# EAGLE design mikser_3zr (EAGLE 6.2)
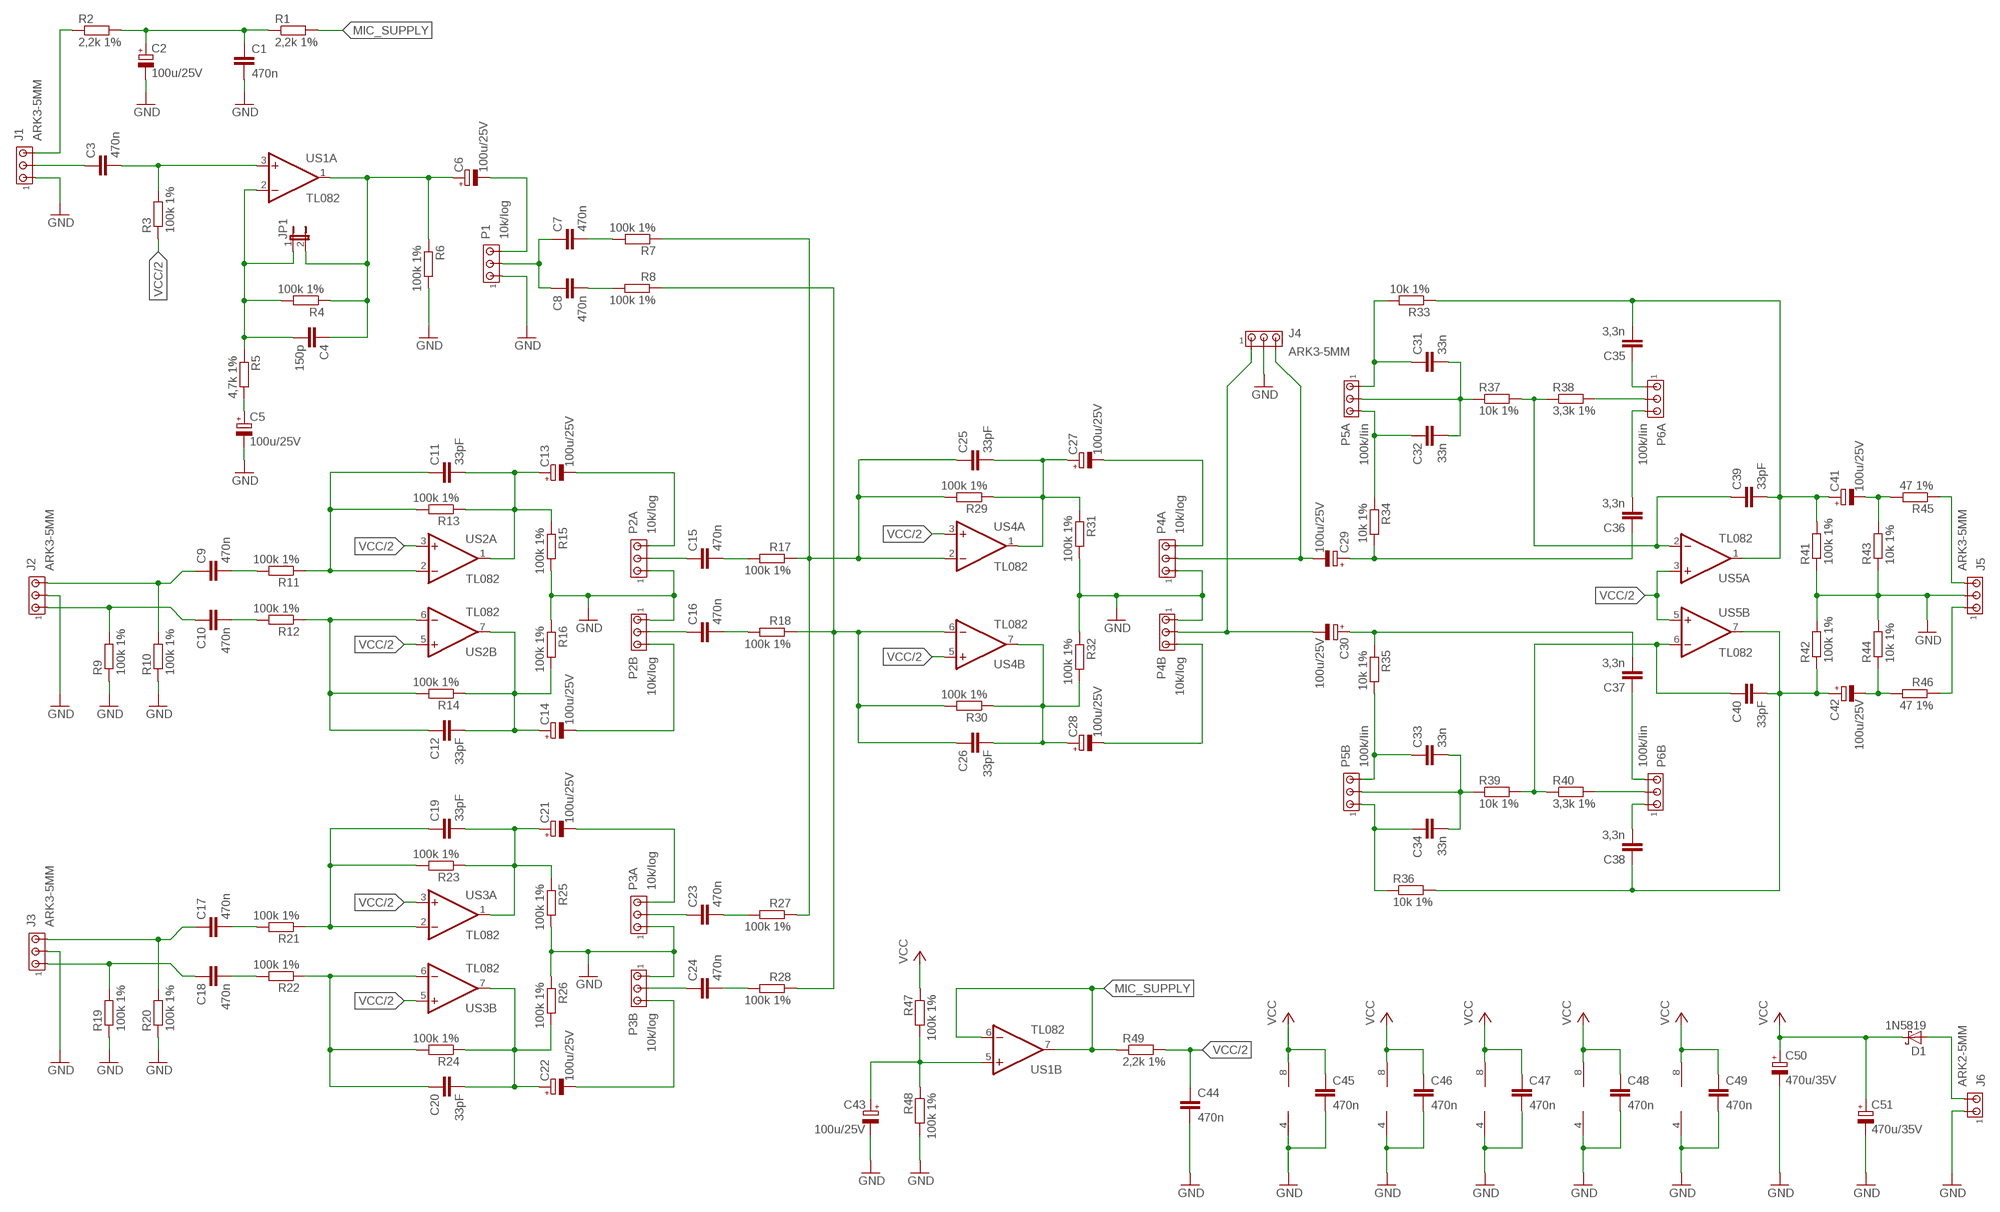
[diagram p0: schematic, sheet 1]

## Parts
C1  470n  C-EU050-055X075  [C050-055X075]
C2  100u/25V  CPOL-EUE2.5-6  [E2,5-6]
C3  470n  C-EU050-055X075  [C050-055X075]
C4  150p  C-EU050-025X075  [C050-025X075]
C5  100u/25V  CPOL-EUE2.5-6  [E2,5-6]
C6  100u/25V  CPOL-EUE2.5-6  [E2,5-6]
C7  470n  C-EU050-055X075  [C050-055X075]
C8  470n  C-EU050-055X075  [C050-055X075]
C9  470n  C-EU050-055X075  [C050-055X075]
C10  470n  C-EU050-055X075  [C050-055X075]
C11  33pF  C-EU050-025X075  [C050-025X075]
C12  33pF  C-EU050-025X075  [C050-025X075]
C13  100u/25V  CPOL-EUE2.5-6  [E2,5-6]
C14  100u/25V  CPOL-EUE2.5-6  [E2,5-6]
C15  470n  C-EU050-055X075  [C050-055X075]
C16  470n  C-EU050-055X075  [C050-055X075]
C17  470n  C-EU050-055X075  [C050-055X075]
C18  470n  C-EU050-055X075  [C050-055X075]
C19  33pF  C-EU050-025X075  [C050-025X075]
C20  33pF  C-EU050-025X075  [C050-025X075]
C21  100u/25V  CPOL-EUE2.5-6  [E2,5-6]
C22  100u/25V  CPOL-EUE2.5-6  [E2,5-6]
C23  470n  C-EU050-055X075  [C050-055X075]
C24  470n  C-EU050-055X075  [C050-055X075]
C25  33pF  C-EU050-025X075  [C050-025X075]
C26  33pF  C-EU050-025X075  [C050-025X075]
C27  100u/25V  CPOL-EUE2.5-6  [E2,5-6]
C28  100u/25V  CPOL-EUE2.5-6  [E2,5-6]
C29  100u/25V  CPOL-EUE2.5-6  [E2,5-6]
C30  100u/25V  CPOL-EUE2.5-6  [E2,5-6]
C31  33n  C-EU050-025X075  [C050-025X075]
C32  33n  C-EU050-025X075  [C050-025X075]
C33  33n  C-EU050-025X075  [C050-025X075]
C34  33n  C-EU050-025X075  [C050-025X075]
C35  3,3n  C-EU050-025X075  [C050-025X075]
C36  3,3n  C-EU050-025X075  [C050-025X075]
C37  3,3n  C-EU050-025X075  [C050-025X075]
C38  3,3n  C-EU050-025X075  [C050-025X075]
C39  33pF  C-EU050-025X075  [C050-025X075]
C40  33pF  C-EU050-025X075  [C050-025X075]
C41  100u/25V  CPOL-EUE2.5-6  [E2,5-6]
C42  100u/25V  CPOL-EUE2.5-6  [E2,5-6]
C43  100u/25V  CPOL-EUE2.5-6  [E2,5-6]
C44  470n  C-EU050-055X075  [C050-055X075]
C45  470n  C-EU050-055X075  [C050-055X075]
C46  470n  C-EU050-055X075  [C050-055X075]
C47  470n  C-EU050-055X075  [C050-055X075]
C48  470n  C-EU050-055X075  [C050-055X075]
C49  470n  C-EU050-055X075  [C050-055X075]
C50  470u/35V  CPOL-EUE5-10.5  [E5-10,5]
C51  470u/35V  CPOL-EUE5-10.5  [E5-10,5]
D1  1N5819  1N5817-B  [DO41-7.6]
J1  ARK3-5MM  [3PIN-5MM]
J2  ARK3-5MM  [3PIN-5MM]
J3  ARK3-5MM  [3PIN-5MM]
J4  ARK3-5MM  [3PIN-5MM]
J5  ARK3-5MM  [3PIN-5MM]
J6  ARK2-5MM  [2PIN-5MM]
JP1  JP1E  [JP1]
P1  10k/log  ARK3-5MM-WASKI  [3PIN-5M-WASKI]
P2A  10k/log  ARK3-5MM-WASKI  [3PIN-5M-WASKI]
P2B  10k/log  ARK3-5MM-WASKI  [3PIN-5M-WASKI]
P3A  10k/log  ARK3-5MM-WASKI  [3PIN-5M-WASKI]
P3B  10k/log  ARK3-5MM-WASKI  [3PIN-5M-WASKI]
P4A  10k/log  ARK3-5MM-WASKI  [3PIN-5M-WASKI]
P4B  10k/log  ARK3-5MM-WASKI  [3PIN-5M-WASKI]
P5A  100k/lin  ARK3-5MM-WASKI  [3PIN-5M-WASKI]
P5B  100k/lin  ARK3-5MM-WASKI  [3PIN-5M-WASKI]
P6A  100k/lin  ARK3-5MM-WASKI  [3PIN-5M-WASKI]
P6B  100k/lin  ARK3-5MM-WASKI  [3PIN-5M-WASKI]
R1  2,2k 1%  R-EU_0207/7  [0207/7]
R2  2,2k 1%  R-EU_0207/7  [0207/7]
R3  100k 1%  R-EU_0207/7  [0207/7]
R4  100k 1%  R-EU_0207/7  [0207/7]
R5  4,7k 1%  R-EU_0207/7  [0207/7]
R6  100k 1%  R-EU_0207/7  [0207/7]
R7  100k 1%  R-EU_0207/7  [0207/7]
R8  100k 1%  R-EU_0207/7  [0207/7]
R9  100k 1%  R-EU_0207/7  [0207/7]
R10  100k 1%  R-EU_0207/7  [0207/7]
R11  100k 1%  R-EU_0207/7  [0207/7]
R12  100k 1%  R-EU_0207/7  [0207/7]
R13  100k 1%  R-EU_0207/7  [0207/7]
R14  100k 1%  R-EU_0207/7  [0207/7]
R15  100k 1%  R-EU_0207/7  [0207/7]
R16  100k 1%  R-EU_0207/7  [0207/7]
R17  100k 1%  R-EU_0207/7  [0207/7]
R18  100k 1%  R-EU_0207/7  [0207/7]
R19  100k 1%  R-EU_0207/7  [0207/7]
R20  100k 1%  R-EU_0207/7  [0207/7]
R21  100k 1%  R-EU_0207/7  [0207/7]
R22  100k 1%  R-EU_0207/7  [0207/7]
R23  100k 1%  R-EU_0207/7  [0207/7]
R24  100k 1%  R-EU_0207/7  [0207/7]
R25  100k 1%  R-EU_0207/7  [0207/7]
R26  100k 1%  R-EU_0207/7  [0207/7]
R27  100k 1%  R-EU_0207/7  [0207/7]
R28  100k 1%  R-EU_0207/7  [0207/7]
R29  100k 1%  R-EU_0207/7  [0207/7]
R30  100k 1%  R-EU_0207/7  [0207/7]
R31  100k 1%  R-EU_0207/7  [0207/7]
R32  100k 1%  R-EU_0207/7  [0207/7]
R33  10k 1%  R-EU_0207/7  [0207/7]
R34  10k 1%  R-EU_0207/7  [0207/7]
R35  10k 1%  R-EU_0207/7  [0207/7]
R36  10k 1%  R-EU_0207/7  [0207/7]
R37  10k 1%  R-EU_0207/7  [0207/7]
R38  3,3k 1%  R-EU_0207/7  [0207/7]
R39  10k 1%  R-EU_0207/7  [0207/7]
R40  3,3k 1%  R-EU_0207/7  [0207/7]
R41  100k 1%  R-EU_0207/7  [0207/7]
R42  100k 1%  R-EU_0207/7  [0207/7]
R43  10k 1%  R-EU_0207/7  [0207/7]
R44  10k 1%  R-EU_0207/7  [0207/7]
R45  47 1%  R-EU_0207/7  [0207/7]
R46  47 1%  R-EU_0207/7  [0207/7]
R47  100k 1%  R-EU_0207/7  [0207/7]
R48  100k 1%  R-EU_0207/7  [0207/7]
R49  2,2k 1%  R-EU_0207/7  [0207/7]
US1  TL082  TL082P  [DIL08]
US2  TL082  TL082P  [DIL08]
US3  TL082  TL082P  [DIL08]
US4  TL082  TL082P  [DIL08]
US5  TL082  TL082P  [DIL08]

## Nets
GND: C1.2 C2.- C5.- C43.- C44.2 C45.2 C46.2 C47.2 C48.2 C49.2 C50.- C51.- J1.P$1 J2.P$2 J3.P$2 J4.P$2 J5.P$2 J6.P$1 P1.P$1 P2A.P$1 P2B.P$1 P3A.P$1 P3B.P$1 P4A.P$1 P4B.P$1 R6.2 R9.1 R10.1 R15.2 R16.1 R19.1 R20.1 R25.2 R26.1 R31.2 R32.1 R41.1 R42.2 R43.1 R44.2 R48.2 US1.4(P:V-) US2.4(P:V-) US3.4(P:V-) US4.4(P:V-) US5.4(P:V-)
MIC_SUPPLY: R1.2 R49.1 US1.6(B:-IN) US1.7(B:OUT)
N$1: J1.P$3 R2.1
N$2: C1.1 C2.+ R1.1 R2.2
N$3: C3.1 J1.P$2
N$4: C3.2 R3.2 US1.3(A:+IN)
N$5: C5.+ R5.2
N$6: C4.2 JP1.1 R4.2 R5.1 US1.2(A:-IN)
N$7: C6.- P1.P$3
N$8: C4.1 C6.+ JP1.2 R4.1 R6.1 US1.1(A:OUT)
N$9: C7.1 C8.1 P1.P$2
N$10: C7.2 R7.2
N$11: C8.2 R8.2
N$12: C10.1 J2.P$1 R9.2
N$13: C9.1 J2.P$3 R10.2
N$14: C9.2 R11.2
N$15: C10.2 R12.2
N$16: C11.2 C13.+ R13.1 R15.1 US2.1(A:OUT)
N$17: C12.2 C14.+ R14.1 R16.2 US2.7(B:OUT)
N$18: C12.1 R12.1 R14.2 US2.6(B:-IN)
N$19: C11.1 R11.1 R13.2 US2.2(A:-IN)
N$20: C13.- P2A.P$3
N$21: C14.- P2B.P$3
N$22: C16.2 R18.2
N$23: C16.1 P2B.P$2
N$24: C15.1 P2A.P$2
N$25: C15.2 R17.2
N$26: C18.1 J3.P$1 R19.2
N$27: C17.1 J3.P$3 R20.2
N$28: C17.2 R21.2
N$29: C18.2 R22.2
N$30: C20.1 R22.1 R24.2 US3.6(B:-IN)
N$31: C19.1 R21.1 R23.2 US3.2(A:-IN)
N$32: C19.2 C21.+ R23.1 R25.1 US3.1(A:OUT)
N$33: C20.2 C22.+ R24.1 R26.2 US3.7(B:OUT)
N$34: C21.- P3A.P$3
N$35: C22.- P3B.P$3
N$36: C24.2 R28.2
N$37: C24.1 P3B.P$2
N$38: C23.1 P3A.P$2
N$39: C23.2 R27.2
N$40: C26.1 R8.1 R18.1 R28.1 R30.2 US4.6(B:-IN)
N$41: C25.1 R7.1 R17.1 R27.1 R29.2 US4.2(A:-IN)
N$42: C25.2 C27.+ R29.1 R31.1 US4.1(A:OUT)
N$43: C26.2 C28.+ R30.1 R32.2 US4.7(B:OUT)
N$44: C27.- P4A.P$3
N$45: C28.- P4B.P$3
N$46: C30.- J4.P$1 P4B.P$2
N$47: C29.- J4.P$3 P4A.P$2
N$48: C29.+ C36.1 R34.2
N$49: C30.+ C37.2 R35.1
N$50: C41.- R43.2 R45.2
N$51: C42.- R44.1 R46.2
N$52: C43.+ R47.2 R48.1 US1.5(B:+IN)
N$53: J5.P$1 R46.1
N$54: J5.P$3 R45.1
N$55: D1.A J6.P$2
N$58: C32.1 P5A.P$3 R34.1
N$59: C31.1 P5A.P$1 R33.2
N$60: C31.2 C32.2 P5A.P$2 R37.1
N$61: C39.1 R37.2 R38.1 US5.2(A:-IN)
N$62: P6A.P$2 R38.2
N$63: C35.2 C39.2 C41.+ R33.1 R41.2 US5.1(A:OUT)
N$65: C33.1 P5B.P$3 R35.2
N$66: C34.1 P5B.P$1 R36.1
N$67: C33.2 C34.2 P5B.P$2 R39.1
N$68: C38.1 C40.2 C42.+ R36.2 R42.1 US5.7(B:OUT)
N$69: C40.1 R39.2 R40.1 US5.6(B:-IN)
N$70: P6B.P$2 R40.2
N$76: C38.2 P6B.P$1
N$77: C37.1 P6B.P$3
N$78: C36.2 P6A.P$3
N$79: C35.1 P6A.P$1
VCC: C45.1 C46.1 C47.1 C48.1 C49.1 C50.+ C51.+ D1.C R47.1 US1.8(P:V+) US2.8(P:V+) US3.8(P:V+) US4.8(P:V+) US5.8(P:V+)
VCC/2: C44.1 R3.1 R49.2 US2.3(A:+IN) US2.5(B:+IN) US3.3(A:+IN) US3.5(B:+IN) US4.3(A:+IN) US4.5(B:+IN) US5.3(A:+IN) US5.5(B:+IN)

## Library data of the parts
C1 C3 C4 C7-C12 C15-C20 C23-C26 C31-C40 C44-C49 = rcl:C-EU: CAPACITOR, European symbol
C2 C5 C6 C13 C14 C21 C22 C27-C30 C41-C43 C50 C51 = rcl:CPOL-EU: POLARIZED CAPACITOR, European symbol
D1 = diode:1N581*: 1.0A SCHOTTKY BARRIER RECTIFIER
J1-J5 P1 P2A P2B P3A P3B P4A P4B P5A P5B P6A P6B = zlacza_futrzak:ARK3: ARK 3 Raster 5mm i 3,5mm
J6 = zlacza_futrzak:ARK2: ARK 2
JP1 = jumper:JP1E: JUMPER
R1-R49 = rcl:R-EU_: RESISTOR, European symbol
US1-US5 = linear:TL082: OP AMP

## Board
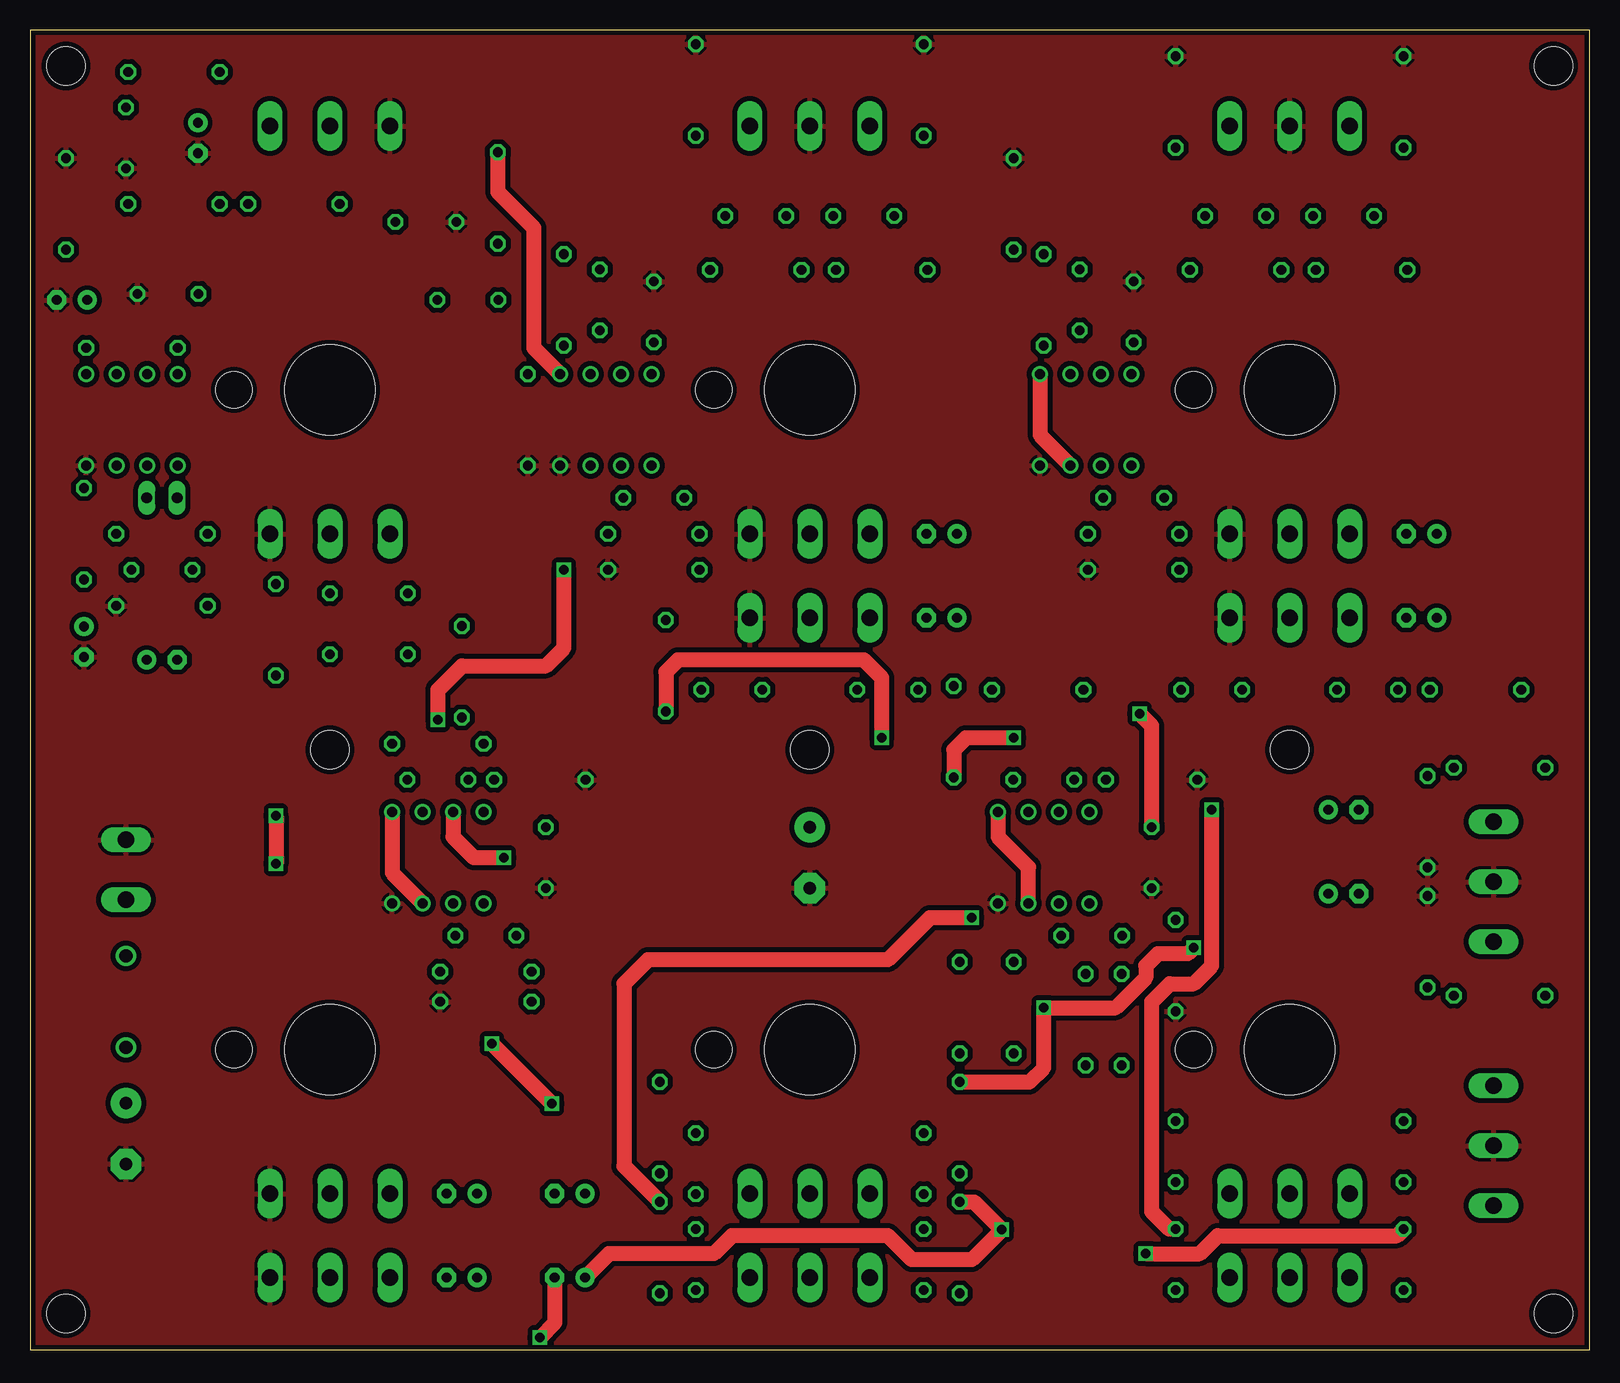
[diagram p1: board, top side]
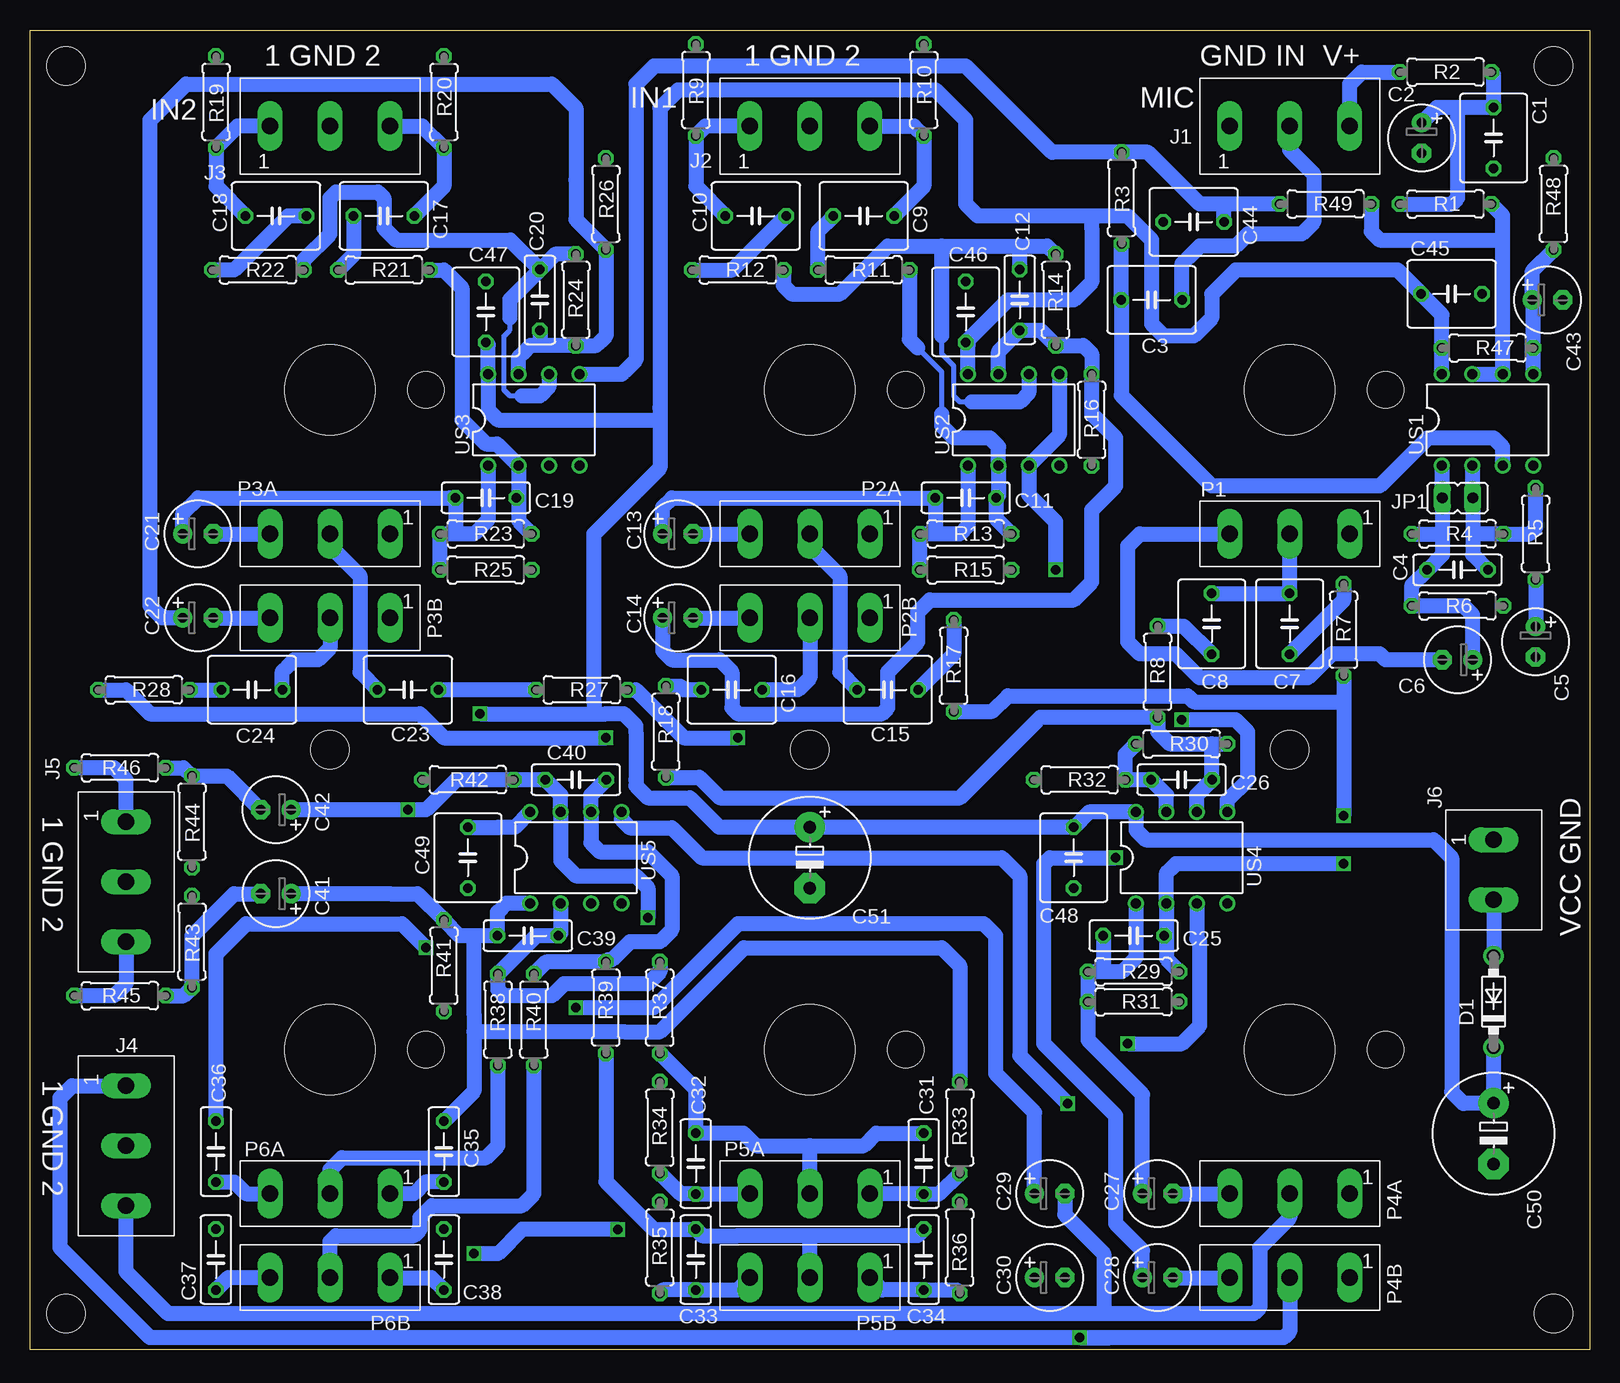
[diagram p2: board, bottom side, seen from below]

Size 130 x 110 mm. Coordinates in mm from the lower left corner, seen from the top.
Outline: 0,0 130,0 130,110 0,110 0,0
Copper layers (1*16): Top 0.035mm / dielectric 1.5mm / Bottom 0.035mm
Design rules: minimum track width 10mil, minimum drill 24mil, track to track 8mil, track to pad 8mil, pad to pad 8mil, via to via 8mil, smd to smd 8mil, copper to edge 10mil, drill to drill 8mil, minimum pad ring 10mil, minimum via ring 8mil, stop-mask expansion 4mil, vias tented up to drill 0mil, thermal gap 10mil
Holes 3.2 mm at 3,3 3,107 127,107 127,3 25,50 65,50 105,50
Holes 7.5 mm at 25,80 65,80 105,80 25,25 65,25 105,25
Holes 3 mm at 17,80 57,80 97,80 17,25 57,25 97,25

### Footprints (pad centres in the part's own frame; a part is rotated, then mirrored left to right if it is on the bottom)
C050-055X075 = drill 0.813 octagon: 1 -2.54,0; 2 2.54,0
E2,5-6 = drill 0.813 pad 1.6: + -1.27,0 | drill 0.813 pad 1.6 octagon: - 1.27,0
C050-025X075 = drill 0.813 octagon: 1 -2.54,0; 2 2.54,0
E5-10,5 = drill 1.016 pad 2.54: + -2.54,0 | drill 1.016 pad 2.54 octagon: - 2.54,0
DO41-7.6 = drill 1.1 pad 1.7: A 3.81,0; C -3.81,0
3PIN-5MM = drill 1.4 long: P$1 -5,0; P$2 0,0; P$3 5,0
2PIN-5MM = drill 1.4 long: P$1 -2.5,0; P$2 2.5,0
JP1 = drill 0.914 long: 1 0,-1.27; 2 0,1.27
3PIN-5M-WASKI = drill 1.4 long: P$1 -5,0; P$2 0,0; P$3 5,0
0207/7 = drill 0.813 octagon: 1 -3.81,0; 2 3.81,0
DIL08 = drill 0.813 pad 1.27: 1 -3.81,-3.81; 2 -1.27,-3.81; 3 1.27,-3.81; 4 3.81,-3.81; 5 3.81,3.81; 6 1.27,3.81; 7 -1.27,3.81; 8 -3.81,3.81

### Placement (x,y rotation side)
C1  8,101 270 bottom
C2  14,101 270 bottom
C3  36.5,87.5 180 bottom
C4  11,65 0 bottom
C5  4.5,59 270 bottom
C6  11,57.5 180 bottom
C7  25,60.5 270 bottom
C8  31.5,60.5 270 bottom
C9  60.5,94.5 180 bottom
C10  69.5,94.5 0 bottom
C11  52,71 180 bottom
C12  47.5,87.5 270 bottom
C13  76,68 0 bottom
C14  76,61 0 bottom
C15  58.5,55 0 bottom
C16  71.5,55 180 bottom
C17  100.5,94.5 180 bottom
C18  109.5,94.5 0 bottom
C19  92,71 180 bottom
C20  87.5,87.5 270 bottom
C21  116,68 0 bottom
C22  116,61 0 bottom
C23  98.5,55 0 bottom
C24  111.5,55 180 bottom
C25  38,34.5 180 bottom
C26  34,47.5 180 bottom
C27  36,13 0 bottom
C28  36,6 0 bottom
C29  45,13 0 bottom
C30  45,6 0 bottom
C31  55.5,15.5 90 bottom
C32  74.5,15.5 90 bottom
C33  74.5,7.5 90 bottom
C34  55.5,7.5 90 bottom
C35  95.5,16.5 90 bottom
C36  114.5,16.5 270 bottom
C37  114.5,7.5 90 bottom
C38  95.5,7.5 270 bottom
C39  88.5,34.5 180 bottom
C40  84.5,47.5 180 bottom
C41  109.5,38 180 bottom
C42  109.5,45 180 bottom
C43  3.5,87.5 0 bottom
C44  33,94 180 bottom
C45  11.5,88 0 bottom
C46  52,86.5 90 bottom
C47  92,86.5 90 bottom
C48  43,41 270 bottom
C49  93.5,41 270 bottom
C50  8,18 270 bottom
C51  65,41 270 bottom
D1  8,29 90 bottom
J1  25,102 0 bottom
J2  65,102 0 bottom
J3  105,102 0 bottom
J4  122,17 270 bottom
J5  122,39 270 bottom
J6  8,40 270 bottom
JP1  11,71 90 bottom
P1  25,68 180 bottom
P2A  65,68 180 bottom
P2B  65,61 180 bottom
P3A  105,68 180 bottom
P3B  105,61 180 bottom
P4A  25,13 180 bottom
P4B  25,6 180 bottom
P5A  65,13 180 bottom
P5B  65,6 180 bottom
P6A  105,13 180 bottom
P6B  105,6 180 bottom
R1  12,95.5 0 bottom
R2  12,106.5 0 bottom
R3  39,96 270 bottom
R4  11,68 0 bottom
R5  4.5,68 270 bottom
R6  11,62 0 bottom
R7  20.5,60 90 bottom
R8  36,56.5 90 bottom
R9  74.5,105 270 bottom
R10  55.5,105 270 bottom
R11  60.5,90 180 bottom
R12  71,90 180 bottom
R13  52,68 0 bottom
R14  44.5,87.5 90 bottom
R15  52,65 0 bottom
R16  41.5,77.5 90 bottom
R17  53,57 90 bottom
R18  77,51.5 90 bottom
R19  114.5,104 270 bottom
R20  95.5,104 270 bottom
R21  100.5,90 180 bottom
R22  111,90 180 bottom
R23  92,68 0 bottom
R24  84.5,87.5 90 bottom
R25  92,65 0 bottom
R26  82,95.5 270 bottom
R27  84,55 180 bottom
R28  120.5,55 0 bottom
R29  38,31.5 0 bottom
R30  34,50.5 0 bottom
R31  38,29 0 bottom
R32  42.5,47.5 0 bottom
R33  52.5,18.5 270 bottom
R34  77.5,18.5 90 bottom
R35  77.5,8.5 270 bottom
R36  52.5,8.5 90 bottom
R37  77.5,28.5 90 bottom
R38  91,27.5 270 bottom
R39  82,28.5 90 bottom
R40  88,27.5 270 bottom
R41  95.5,32 90 bottom
R42  93.5,47.5 180 bottom
R43  116.5,34 270 bottom
R44  116.5,44 270 bottom
R45  122.5,29.5 0 bottom
R46  122.5,48.5 0 bottom
R47  8.5,83.5 0 bottom
R48  3,95.5 90 bottom
R49  22,95.5 180 bottom
US1  8.5,77.5 0 bottom
US2  48,77.5 0 bottom
US3  88,77.5 0 bottom
US4  34,41 0 bottom
US5  84.5,41 0 bottom

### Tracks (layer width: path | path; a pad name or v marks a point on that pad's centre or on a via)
GND
  pour Top (isolate 0.406): 0,0 130,0 130,110 0,110
MIC_SUPPLY
  Bottom 1.27: US1.7 US1.6 7.23,92.5 | 7.23,92.5 7.23,94.54 R1.2 | R49.1 18.19,93.19 17.5,92.5 7.23,92.5
N$1
  Bottom 1.27: J1.P$3 20,105.5 19,106.5 R2.1
N$2
  Bottom 1.27: 11,103.54 C1.1 8,106.31 R2.2 | 11,103.54 12.73,103.54 C2.+ | R1.1 11.5,95.5 11,96 11,103.54
N$3
  Bottom 1.27: J1.P$2 25,100 23,98 23,94 24,93 28.5,93 29.5,92 32.5,92 33.5,91 33.96,90.54 C3.1
N$4
  Bottom 1.27: R3.2 39.04,92.15 C3.2 39.04,79.54 31.5,72 17.5,72 13.5,76 8,76 7.23,75.23 US1.3
N$5
  Bottom 1.27: R5.2 C5.+
N$6
  Bottom 1.27: US1.2 9.77,71.04 JP1.1 9.73,68 | 9.73,68 9.73,66.27 C4.2 | 9.73,68 R4.2 5,68 4.5,68.5 R5.1
N$7
  Bottom 1.27: C6.- 17,57.5 17.5,58 21.5,58 23,56.5 23.5,56 32.5,56 34.5,58 37.5,58 38.5,59 38.5,67 37.5,68 P1.P$3
N$8
  Bottom 1.27: US1.1 12.31,71.04 JP1.2 12.27,68 | 12.27,68 12.27,66.27 C4.1 14.81,63.73 R6.1 10.5,62 9.73,61.23 C6.+ | R4.1 12.27,68
N$9
  Bottom 1.27: C8.1 C7.1 P1.P$2
N$10
  Bottom 1.27: R7.2 20.5,62.46 C7.2
N$11
  Bottom 1.27: R8.2 33.85,60.31 C8.2
N$12
  Bottom 1.27: J2.P$1 73.69,102 R9.2 74.5,96.96 C10.1
N$13
  Bottom 1.27: J2.P$3 56.31,102 R10.2 55.5,96.96 C9.1
N$14
  Bottom 1.27: R11.2 64.31,93.23 C9.2
N$15
  Bottom 1.27: R12.2 71.46,90 C10.2
N$16
  Bottom 1.27: US2.1 51.81,68.69 52.5,68 54.5,68 | 54.5,68 R13.1 R15.1 | 54.5,68 54.54,68.04 C11.2 76.5,71 77.27,70.23 C13.+
N$17
  Bottom 1.27: US2.7 49.27,83.19 C12.2 45.77,84.96 R14.1 42.19,83.69 41.5,83 R16.2 41.5,78 39.5,76 39.5,72 41.5,70 41.5,64 43,62.5 55,62.5 56,61.5 56,59 58.5,56.5 58.5,53.5 59,53 71,53 71.5,53.5 71.5,56.5 72.5,57.5 76.5,57.5 77.27,58.27 C14.+
N$18
  Bottom 0.406: 51.5,79 52.5,79 53,79.5 53,82 53.5,82.5 54,83 54,84.5
  Bottom 1.27: R12.1 67.19,88.69 66.5,88 62.5,88 58.5,92 54,92 | 54,92 47.5,92 | 47.5,92 45.19,92 R14.2 | C12.1 47.5,92 | US2.6 46.73,79.77 47.5,79 51.5,79 | 54,84.5 54,92
N$19
  Bottom 0.406: 54,78 54,81.5 56,83.5
  Bottom 1.27: R13.2 49.46,69.27 C11.1 49.27,71.19 US2.2 49.27,75.27 50,76 53,76 54,77 54,78 | R11.1 56.69,84.19 56,83.5
N$20
  Bottom 1.27: C13.- P2A.P$3
N$21
  Bottom 1.27: C14.- P2B.P$3
N$22
  Bottom 1.27: C16.2 75.5,55 75.81,55.31 R18.2
N$23
  Bottom 1.27: P2B.P$2 65,56 66,55 C16.1
N$24
  Bottom 1.27: P2A.P$2 65,67 62.5,64.5 62.5,56.46 C15.1
N$25
  Bottom 1.27: R17.2 53,57.96 C15.2
N$26
  Bottom 1.27: J3.P$1 112.69,102 R19.2 114.5,96.96 C18.1
N$27
  Bottom 1.27: J3.P$3 97.31,102 R20.2 95.5,96.96 C17.1
N$28
  Bottom 1.27: C17.2 103.04,91.27 R21.2
N$29
  Bottom 1.27: C18.2 108.5,94.5 113,90 R22.2
N$30
  Bottom 0.406: 89,79.5 90,79.5 90.5,80 90.5,84.5 90,85 90,86
  Bottom 1.27: R24.2 86.23,91.31 C20.1 | US3.6 86.73,80.27 87.5,79.5 89,79.5 | 90,86 90,87.54 C20.1 | R22.1 107.19,90.81 105,93 105,96 104.5,96.5 101,96.5 100.5,96 100.5,93.5 99.5,92.5 89.96,92.5 C20.1
N$31
  Bottom 1.27: R21.1 95.5,90 94.5,89 94,88.5 94,77.5 92.5,76 92,75.5 91.08,75.5 US3.2 89.27,71 | 89.27,71 89.27,69.08 R23.2 | C19.1 89.27,71
N$32
  Bottom 1.27: US3.1 91.81,69.19 93,68 94.5,68 | 94.5,68 R23.1 R25.1 | 94.5,68 94.54,68.04 C19.2 95,71 116,71 117.27,69.73 C21.+
N$33
  Bottom 1.27: 87.5,83.69 R24.1 82.81,83.69 82.5,84 82,84.5 R26.2 84.5,94.19 84.5,97.5 84.5,103.5 86.5,105.5 117,105.5 117.5,105 120,102.5 120,62 119,61 C22.+ | 87.5,83.69 88.31,83.69 89,83 89.27,82.73 US3.7 | C20.2 87.5,83.69
N$34
  Bottom 1.27: C21.- P3A.P$3
N$35
  Bottom 1.27: C22.- P3B.P$3
N$36
  Bottom 1.27: R28.2 C24.2
N$37
  Bottom 1.27: P3B.P$2 105,58.5 106,57.5 108,57.5 108.5,57 108.96,56.54 C24.1
N$38
  Bottom 1.27: P3A.P$2 105,67 103,65 102.5,64.5 102.5,56.46 C23.1
N$39
  Bottom 1.27: R27.2 C23.2
N$40  (via drill 0.8)
  Top 1.27: v82,51 78,51 77,50 R18.1
  Bottom 1.27: R28.1 122,55 120,53 97.5,53 96.5,52 95.5,51 v82,51 | US4.6 32.73,46.23 C26.1 31.46,50.46 31.5,50.5 | 31.5,50.5 35,50.5 36,51.5 R8.1 45.81,52.69 46,52.5 52.5,46 72.5,46 73,46.5 74.19,47.69 R18.1 | 31.5,50.5 R30.2
N$41  (via drill 0.8)
  Top 1.27: v20.5,44.5 v20.5,40.5 | v71,51 71,56 69.5,57.5 54,57.5 53,56.5 R17.1
  Bottom 1.27: 35.27,34.5 US4.2 35.27,39.73 35,40 34.5,40.5 21.5,40.5 v20.5,40.5 | 35.27,34.5 35.27,32.58 R29.2 | C25.1 35.27,34.5 | R7.1 20.5,54 | 20.5,54 v20.5,44.5 | R17.1 49.81,53.19 48.5,54.5 33.5,54.5 33,54 20.5,54 | R27.1 79.5,55 77,52.5 75.5,51 v71,51
N$42
  Bottom 1.27: US4.1 37.81,32.69 39,31.5 40.5,31.5 | 40.5,31.5 R29.1 R31.1 41.81,25.81 38,22 37.27,21.27 C27.+ | C25.2 40.54,31.54 40.5,31.5
N$43  (via drill 0.8)
  Top 1.27: v39.5,41 37,41 35.5,42.5 35.27,42.73 US4.7
  Bottom 1.27: US4.7 35.27,46.23 C26.2 R32.2 38.69,49.62 R30.1 | C28.+ 37.27,8.27 39,10 39.5,10.5 39.5,16.5 39.5,19.5 44,24 45.5,25.5 45.5,40.5 45,41 v39.5,41
N$44
  Bottom 1.27: C27.- P4A.P$3
N$45
  Bottom 1.27: C28.- P4B.P$3
N$46  (via drill 0.8)
  Top 1.27: C30.- 43.73,2.23 v42.5,1
  Bottom 1.27: P4B.P$2 25,1.5 25.5,1 39,1 40,1 | 40,1 v42.5,1 | v42.5,1 120,1 127.5,8.5 127.5,21 126.5,22 J4.P$1 | v42.5,1 40,1
N$47
  Bottom 1.27: P4A.P$2 25,11 27.5,8.5 27.5,3.5 28,3 32.5,3 40.5,3 | 40.5,3 118.5,3 122,6.5 J4.P$3 | C29.- 43.73,11.23 40.5,8 40.5,3
N$48  (via drill 0.8)
  Top 1.27: R34.2 83.31,22.31 84.5,23.5 v84.5,28.5 90.5,28.5 93,31 93,32 94,33 96.5,33 v97,33.5
  Bottom 1.27: C29.+ 46.27,19.77 48.5,22 48.81,22.31 49.5,23 49.5,34.5 50.5,35.5 71,35.5 78,28.5 82.5,28.5 v84.5,28.5 | C36.1 114.5,33 112,35.5 99,35.5 v97,33.5
N$49  (via drill 0.8)
  Top 1.27: C30.+ 48.27,8 53.5,8 57,8 58.5,9.5 71.5,9.5 73.5,7.5 78.5,7.5 v81,10 78.69,12.31 R35.1 | v93,8 97.5,8 99,9.5 113.96,9.5 C37.2
  Bottom 1.27: v81,10 81.04,10.04 88.96,10.04 91,8 v93,8
N$50
  Bottom 1.27: R45.2 117.19,29.5 R43.2 116.5,34.5 113,38 C41.-
N$51
  Bottom 1.27: R46.2 117.19,48.5 R44.1 113.58,47.81 C42.-
N$52
  Bottom 1.27: R48.1 4.77,89.92 C43.+ 4.69,87.42 R47.2 US1.5
N$53
  Bottom 1.27: J5.P$1 122,47.5 123,48.5 R46.1
N$54
  Bottom 1.27: J5.P$3 122,30.5 123,29.5 R45.1
N$55
  Bottom 1.27: J6.P$2 D1.A
N$58
  Bottom 1.27: P5A.P$3 70.04,12.96 C32.1 75.77,12.96 R34.1
N$59
  Bottom 1.27: P5A.P$1 59.96,12.96 C31.1 54.23,12.96 R33.2
N$60
  Bottom 1.27: 65,17 69.5,17 70.54,18.04 C32.2 74.5,21.69 R37.1 | 65,17 60.5,17 59.46,18.04 C31.2 | P5A.P$2 65,17
N$61
  Bottom 1.27: US5.2 85.77,34.69 C39.1 87.81,34.5 R38.1 91,30 90.5,29.5 86.5,29.5 85.5,30.5 78.5,30.5 77.5,31.5 R37.2
N$62
  Bottom 1.27: P6A.P$2 105,15 104,16 92,16 91,17 R38.2
N$63
  Bottom 1.27: C41.+ 100,38 97.69,38 R41.2 94.19,34.5 93,34.5 | US5.1 90.31,37.19 91,36.5 91.04,36.46 C39.2 93,34.5 | 93,34.5 93,28 93,26.5 | R33.1 52.5,32 54,33.5 70.5,33.5 77.5,26.5 80.5,26.5 91.5,26.5 93,26.5 | 93,26.5 93,21.54 C35.2
N$65
  Bottom 1.27: P5B.P$3 71.04,4.96 C33.1 77.23,4.96 R35.2
N$66
  Bottom 1.27: P5B.P$1 58.96,4.96 C34.1 52.77,4.96 R36.1
N$67
  Bottom 1.27: 65,9.5 56,9.5 56,9.54 C34.2 | 65,9.5 71,9.5 74,9.5 74,9.54 C33.2 78.04,10.04 78.5,10.5 82,14 R39.1 | P5B.P$2 65,9.5
N$68  (via drill 0.8)
  Top 1.27: v78.5,36 75,36 71.5,32.5 51.5,32.5 49.5,30.5 49.5,15.31 R36.2 | C38.1 94.96,10.04 93.5,11.5 93.5,29 95,30.5 97,30.5 98.5,32 v98.5,45
  Bottom 1.27: v98.5,45 97,45 94.5,47.5 R42.1 C40.2 85.77,46.23 US5.7 85.77,40.77 84.5,39.5 79.5,39.5 78.5,38.5 v78.5,36 | v98.5,45 100.5,45 | 100.5,45 C42.+ | v98.5,45 100.5,45
N$69
  Bottom 1.27: C40.1 83.23,46.23 US5.6 83.23,42.23 82.5,41.5 78.5,41.5 76.5,39.5 76.5,35 77.5,34 80,34 81.5,32.5 81.81,32.5 R39.2 87,32.31 R40.1
N$70
  Bottom 1.27: P6B.P$2 105,9 104.5,9.5 98,9.5 97.5,10 97.5,11 96.5,12 89,12 88,13 R40.2
N$76
  Bottom 1.27: P6B.P$1 96.54,6 C38.2
N$77
  Bottom 1.27: P6B.P$3 113.46,6 C37.1
N$78
  Bottom 1.27: C36.2 112.96,13.96 112,13 P6A.P$3
N$79
  Bottom 1.27: C35.1 97.04,13.96 98,13 P6A.P$1
VCC  (via drill 0.8)
  Top 1.27: C49.1 93.5,52 v92.5,53
  Bottom 1.27: US1.8 R47.1 12.31,86.27 C45.1 14.04,88.04 15,89 16,90 29.5,90 31.5,88 31.5,86 33,84.5 35.5,84.5 36.5,85.5 36.5,92.5 38.5,94.5 40.5,94.5 41.5,94.5 | 41.5,94.5 51,94.5 52,95.5 52,102.5 54.5,105 76,105 77.5,103.5 77.5,78.5 77.5,77.5 | 77.5,77.5 77.5,73.5 79.5,71.5 83,68 83,54 83,53 | 41.5,94.5 41.5,93.5 41.5,89 42.5,88 43,87.5 48.46,87.5 C46.1 51.81,83.77 US2.8 | C47.1 91.81,83.77 US3.8 91.81,78.31 91,77.5 77.5,77.5 | D1.C C50.+ 10.46,20.54 10.5,20.5 11.5,21.5 11.5,41 13,42.5 37,42.5 37.81,43.31 US4.8 41.73,44.81 C48.1 C51.+ 71.54,43.54 72.54,43.54 75,46 78.5,46 79.5,47 79.5,47.5 79.5,51.5 79.5,52 80.5,53 82,53 83,53 | US5.8 89.58,43.54 90.96,43.54 91,43.5 93.46,43.5 C49.1 | v92.5,53 83,53
VCC/2  (via drill 0.8)
  Top 1.27: US2.5 42,83.5 42,93.5 39,96.5 R3.1 | US3.5 84.19,76.23 US3.3 | US4.5 30.19,39.73 US4.3 | v34,52.5 34,55 36,57 43,57 44.5,58.5 v44.5,65 | US5.5 80.69,42.73 83.23,40.19 US5.3 | v43.5,20.5 v38.5,25.5
  Bottom 1.27: R49.2 30.5,95.5 | 30.5,95.5 32.5,95.5 36.5,99.5 36.81,99.81 R3.1 44.81,99.81 51.5,106.5 52,107 78,107 79.5,105.5 79.5,82.5 80.5,81.5 80.69,81.31 US3.5 | C44.1 30.46,95.46 30.5,95.5 | US2.5 44.19,76.23 US2.3 46.73,71.23 44.5,69 v44.5,65 | US4.5 30.19,45.81 28.5,47.5 28.5,51.5 29.5,52.5 33.5,52.5 v34,52.5 | US5.5 80.69,44.19 80,43.5 76.5,43.5 74,41 49,41 47.5,39.5 47.5,24.5 v43.5,20.5 | v38.5,25.5 34,25.5 32.5,27 32.5,34 32.73,34.23 US4.3

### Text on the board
bPlace: GND IN V+ | 1 GND 2 | 1 GND 2 | MIC | IN1 | IN2 | VCC GND | 1 GND 2 | 1 GND 2
tStop: INPUT 1 | INPUT 2 | MICROPHONE | Futrzaczek | VOLUME | BASS | TREBLE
